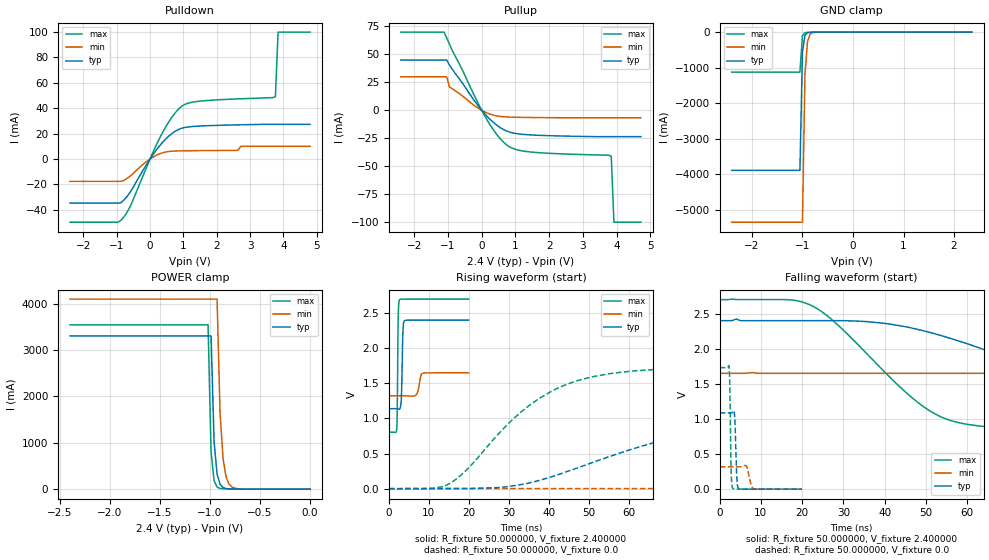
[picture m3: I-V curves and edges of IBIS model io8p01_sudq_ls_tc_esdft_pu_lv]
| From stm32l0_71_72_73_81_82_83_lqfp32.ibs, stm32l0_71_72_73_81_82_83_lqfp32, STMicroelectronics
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|   Model io8p01_sudq_ls_tc_esdft_pu_lv
[Model]  io8p01_sudq_ls_tc_esdft_pu_lv
Model_type I/O
Polarity   Non-Inverting
Enable   Active-Low
Vinl =   0.720000V
Vinh =   1.680000V
Vmeas =  1.200000V
Cref =   50.000000pF
Rref =   100.000000M
Vref =   0.0V
C_comp   2.242700pF   2.201100pF   2.288600pF
[Temperature Range]   25.000000   0.105000k   -40.000000
[Pullup Reference]   2.400000V   1.650000V   2.700000V
[Pulldown Reference]   0.0V   0.0V   0.0V
[POWER Clamp Reference]   2.400000V   1.650000V   2.700000V
[GND Clamp Reference]   0.0V   0.0V   0.0V
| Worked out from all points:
|   slope of the pulldown table from 0 to 0.36 V, typ, clamps not added: 28.4 ohm
|   slope of the pullup table from 0 to 0.36 V, typ, clamps not added: 32.2 ohm
|   GND clamp passes 1 mA (typ) near -0.65 V on its own axis
|   POWER clamp passes 1 mA (typ) near -0.63 V on its own axis
|   rising waveform, R_fixture 50.000000, V_fixture 2.400000: 20-80 % time 278ps typ, 629ps min, 186ps max; typ from 1.14 V to 2.4 V
|   rising waveform, R_fixture 50.000000, V_fixture 0.0: 20-80 % time 40.6ns typ, 109ns min, 19.8ns max; typ from 0.001 V to 1.09 V
|   falling waveform, R_fixture 50.000000, V_fixture 2.400000: 20-80 % time 41.3ns typ, 105ns min, 20.3ns max; typ from 2.4 V to 1.14 V
|   falling waveform, R_fixture 50.000000, V_fixture 0.0: 20-80 % time 354ps typ, 755ps min, 262ps max; typ from 1.09 V to 0.001 V
[Pulldown]
|Voltage   I(typ)   I(min)   I(max)
-2.4V     -34.71mA   -17.61mA   -49.77mA
-880mV    -34.55mA   -17.61mA   -48.41mA
-560mV    -24.66mA   -12.69mA   -35.31mA
240mV     8.893mA    3.542mA    13.9mA
560mV     17.98mA    5.931mA    29.16mA
880mV     23.58mA    6.388mA    40.03mA
1.44V     25.89mA    6.593mA    45.41mA
2.64V     26.92mA    7mA        47.38mA
2.72V     26.96mA    10mA       47.46mA
3.76V     27.3mA     10mA       49mA
3.84V     27.3mA     10mA       100mA
4.8V      27.3mA     10mA       100mA
[Pullup]
|Voltage   I(typ)   I(min)   I(max)
-2.4V     45mA       30mA       70mA
-1.12V    45mA       30mA       70mA
-1.04V    45mA       30mA       64.8mA
-960mV    40.7mA     21mA       59.3mA
80mV      -2.838mA   -1.261mA   -4.478mA
480mV     -14.04mA   -5.167mA   -22.91mA
800mV     -19.2mA    -5.978mA   -32.18mA
1.04V     -20.85mA   -6.184mA   -35.23mA
1.44V     -21.93mA   -6.373mA   -37.19mA
3.84V     -23.5mA    -6.63mA    -41mA
3.92V     -23.5mA    -6.63mA    -100mA
4.72V     -23.5mA    -6.63mA    -100mA
[GND_clamp]
|Voltage   I(typ)   I(min)   I(max)
-2.4V     -3.892A    -5.353A    -1.127A
-1.05V    -3.892A    -5.353A    -1.127A
-1V       -568.8mA   -5.353A    -105.4mA
-950mV    -88.95mA   -1.19A     -18.03mA
-900mV    -18.15mA   -269.2mA   -8.959mA
-850mV    -6.699mA   -63.45mA   -6.568mA
-800mV    -4.014mA   -16.61mA   -4.858mA
-650mV    -1.043mA   -1.218mA   -1.146mA
2.35V     0A         0A         0A
[POWER_clamp]
|Voltage   I(typ)   I(min)   I(max)
-2.4V     3.303A     4.097A     3.542A
-1.02V    3.303A     4.097A     3.542A
-990mV    3.303A     4.097A     802.4mA
-960mV    1.032A     4.097A     186.5mA
-930mV    325.2mA    4.097A     47.6mA
-900mV    104.9mA    1.637A     15.79mA
-870mV    35.84mA    655.7mA    8.024mA
-840mV    13.94mA    263.9mA    5.676mA
-810mV    6.724mA    107.2mA    4.568mA
-780mV    4.1mA      44.41mA    3.772mA
-690mV    1.753mA    4.377mA    1.918mA
0V        0A         0A         0A
[Ramp]
| variable   typ   min   max
dV/dt_r  0.65100/40.55304n   0.19006/0.10913u   1.03799/19.79288n
dV/dt_f  0.75624/41.27034n   0.19440/0.10539u   1.13750/20.23202n
R_load = 50.000000
[Rising Waveform]
R_fixture= 50.000000
V_fixture= 2.400000
V_fixture_min= 1.650000
V_fixture_max= 2.700000
|time   V(typ)   V(min)   V(max)
0s        1.14V      1.322V     804.2mV
1.962ns   1.14V      1.322V     846.2mV
2.082ns   1.139V     1.322V     1.037V
2.322ns   1.135V     1.322V     2.398V
2.683ns   1.134V     1.322V     2.69V
3.123ns   1.296V     1.323V     2.699V
3.483ns   2.192V     1.323V     2.699V
3.844ns   2.388V     1.323V     2.7V
8.488ns   2.4V       1.643V     2.7V
19.94ns   2.4V       1.65V      2.7V
[Rising Waveform]
R_fixture= 50.000000
V_fixture= 0.0
V_fixture_min= 0.0
V_fixture_max= 0.0
|time   V(typ)   V(min)   V(max)
0s        892uV      1.338mV    523.9uV
15.02ns   2.536mV    2.497mV    68.64mV
33.03ns   59.45mV    2.498mV    1.092V
43.04ns   215mV      2.498mV    1.453V
52.05ns   396.5mV    2.502mV    1.606V
67.07ns   668.2mV    2.637mV    1.699V
95.1ns    952.5mV    4.12mV     1.728V
139.1ns   1.069V     50.88mV    1.73V
278.3ns   1.086V     276.2mV    1.73V
498.5ns   1.086V     318.6mV    1.73V
[Falling Waveform]
R_fixture= 50.000000
V_fixture= 2.400000
V_fixture_min= 1.650000
V_fixture_max= 2.700000
|time   V(typ)   V(min)   V(max)
0s        2.4V       1.65V      2.7V
22.02ns   2.4V       1.65V      2.622V
36.04ns   2.385V     1.65V      1.909V
51.05ns   2.231V     1.65V      1.112V
58.06ns   2.109V     1.65V      946.9mV
69.07ns   1.884V     1.65V      866.9mV
99.1ns    1.372V     1.65V      816.6mV
134.1ns   1.208V     1.639V     806.5mV
282.3ns   1.14V      1.388V     804.2mV
498.5ns   1.14V      1.322V     804.2mV
[Falling Waveform]
R_fixture= 50.000000
V_fixture= 0.0
V_fixture_min= 0.0
V_fixture_max= 0.0
|time   V(typ)   V(min)   V(max)
0s        1.086V     318.6mV    1.73V
2.282ns   1.086V     318.6mV    1.748V
2.442ns   1.086V     318.6mV    1.497V
2.763ns   1.085V     318.6mV    287.5mV
3.163ns   1.098V     318.6mV    14.03mV
3.604ns   1.057V     318.6mV    1.025mV
4.164ns   152.6mV    318.4mV    517.2uV
4.605ns   8.627mV    318.1mV    522.3uV
8.248ns   889uV      7.026mV    526.4uV
19.94ns   892uV      1.338mV    523.9uV
